(* Logix 5000 AddOnInstructionDefinition export Banner_S15C_MGN_Param_v4; software revision 33.00 *)

TYPE Banner_IOL_Port_v4 :   // UDT that has all of the data items necessary to communicate with a specific Port on a IO-Link Master
STRUCT
   Port_Controlled : INT;   // Each bit represents a port on an IO-Link Master. Set to 1 to tell AOI to control that port.
   Port_Activate : INT;   // Each bit represents a port on an IO-Link Master. When ON that port will process any commands in queue.
   Port_Read : INT;   // Each bit represents a port on an IO-Link Master. Used to determine when device AOI has requested a Read command.
   Port_Write : INT;   // Each bit represents a port on an IO-Link Master. Used to determine when device AOI has requested a Write command.
   Port_RW_Complete : INT;   // Each bit represents a port on an IO-Link Master. Tells device AOI that Read or Write request has been completed.
   Port_Device_Read : INT;
   Data_Transfer : SINT[190];   // Array to transfer data from IO-Master to device AOIs.
END_STRUCT
END_TYPE

TYPE Banner_S15C_MGN_RD_v4 :   // All of the read parameters for a S15C.
STRUCT
   Master_Cycle_Time : INT;
   Min_Cycle_Time : INT;
   M_Sequence_Capability : INT;
   IO_Link_Version_ID : INT;
   Process_Data_Input_Length : INT;
   Process_Data_Output_Length : INT;
   Combined_Vendor_ID : DINT;   // IO-Link Vendor ID
   Vendor_ID1 : INT;
   Vendor_ID2 : INT;
   Combined_Device_ID : DINT;   // IO-Link Device ID
   Device_ID1 : INT;
   Device_ID2 : INT;
   Device_ID3 : INT;
   Serial_Number : STRING;
   Product_Name : STRING;
END_STRUCT
END_TYPE

TYPE Banner_S15C_MGN_v4 :   // All of the parameters for a S15C.
STRUCT
   Initial_Global_Read : BOOL;   // Determines if all of the IO-Link data has been read into the PLC yet
   Command : INT;   // Value placed in here will activate a read or write to a specifc IO-Link Index
   Read : Banner_S15C_MGN_RD_v4;   // Read Only Data
   Write : Banner_S15C_MGN_WD_v4;   // Write Data
   Archive : Banner_S15C_MGN_WD_v4;   // Archive Data
   Reset : BOOL;   // Resets AOI. This will force a complete parameter read of the sensor.
END_STRUCT
END_TYPE

TYPE Banner_S15C_MGN_WD_v4 :   // UDT that stores the Write Data for a S15C.
STRUCT
   System_Command : INT;   // See IODD file for list of commands that can be activated via the System Command interface
   Parameter_Access_Lock : SINT;   // Write access to all parameters is prohibited while value is 1. Only this parameter can be adjusted when value is 1.
   Data_Storage_Lock : SINT;   // Automatic data storage is disabled when this value is equal to 1. Read access is not affected.
   Local_Parameterization_Lock : SINT;   // Parameterization via local control elements on device is disabled.
   Local_User_Interface_Lock : SINT;   // Operation of local user interface is disabled.
   Modbus_Address : DINT;   // 0 to 255
   Modbus_Baud_Rate : DINT;   // 1 to 65535
   Modbus_Parity : DINT;   // 0 to 2
   Modbus_Stop_Bits : DINT;   // 0 to 2
   Modbus_Compliance_Mode : DINT;   // 0 to 4
   RRS : Banner_S15C_RRSS_v4[4];   // Read Register Sets
   WRS : Banner_S15C_WRSS_v4[16];   // Write Registers Set
END_STRUCT
END_TYPE

TYPE Banner_S15C_RRSS_v4 :   // Read Register Set Settings
STRUCT
   MB_Reg : DINT[16];   // Index 1 through 15 are used to store the Modbus Registers
END_STRUCT
END_TYPE

TYPE Banner_S15C_WRSS_v4 :   // Write Register Set Settings
STRUCT
   MB_Reg : DINT;   // Index 1 through 15 are used to store the Modbus registers
   MB_Update_Type : SINT;   // Index 1 through 15 used to store the Modbus registers update type
   MB_Check_Result : SINT;   // Index 1 through 15 used to store the Modbus Check Result
   MB_Write_Cmd_Type : SINT;   // Index 1 through 15 used to store the Write Command type
END_STRUCT
END_TYPE

ADD_ON_INSTRUCTION Banner_S15C_MGN_Param_v4   (* revision 4.0, vendor Banner Engineering *)
// AOI to read and write parameter data to an IO-Link S15C.
VAR_IN_OUT
   S15C : Banner_S15C_MGN_v4; {required}
   Port_Data : Banner_IOL_Port_v4; {required}
END_VAR
VAR_INPUT
   Port : DINT; {required}
END_VAR
VAR
   Local_Control : DINT; {access None}
   Global_Read_Command_Value : INT; {access None}
   Global_Write_Command_Value : INT; {access None}
   Error_Generated : BOOL; {access None}
   Command_Being_Processed : BOOL; {access None}
   Index_Write_Inprocess : INT; {access None}
   Index_Write_Control : INT; {access None}
   Update_Archive : BOOL; {access None}
   Inprocess_Index : DINT; {access None}
   RRS_Index0 : SINT; {access None}
   WRS_Index1 : SINT; {access None}
   WRS_Index0 : SINT; {access None}
   RRS_Index2 : SINT; {access None}
   RRS_Index1 : SINT; {access None}
   RRS_Index3 : SINT; {access None}
   WRS_Index2 : SINT; {access None}
   WRS_Index3 : SINT; {access None}
   WRS_Index4 : SINT; {access None}
   DoNotRun : BOOL; {access None}
   WR_Control : DINT; {access None}
END_VAR

ROUTINE Logic   (* ladder *)
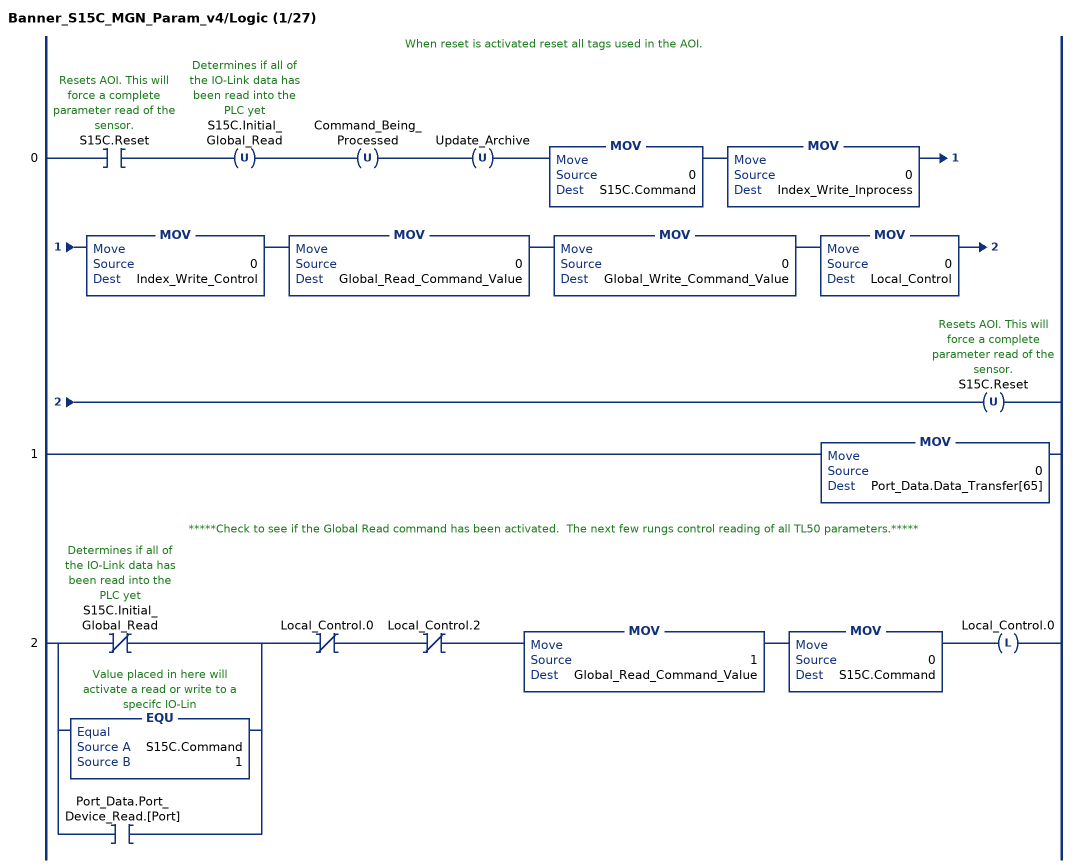
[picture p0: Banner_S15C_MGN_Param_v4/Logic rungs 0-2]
   // When reset is activated reset all tags used in the AOI.
   0: XIC(S15C.Reset)OTU(S15C.Initial_Global_Read)OTU(Command_Being_Processed)OTU(Update_Archive)MOV(0,S15C.Command)MOV(0,Index_Write_Inprocess)MOV(0,Index_Write_Control)MOV(0,Global_Read_Command_Value)MOV(0,Global_Write_Command_Value)MOV(0,Local_Control)OTU(S15C.Reset);
   1: MOV(0,Port_Data.Data_Transfer[65]);
   // *****Check to see if the Global Read command has been activated.  The next few rungs control reading of all TL50 parameters.*****
   2: [XIO(S15C.Initial_Global_Read) ,EQU(S15C.Command,1) ,XIC(Port_Data.Port_Device_Read.[Port]) ]XIO(Local_Control.0)XIO(Local_Control.2)MOV(1,Global_Read_Command_Value)MOV(0,S15C.Command)OTL(Local_Control.0);
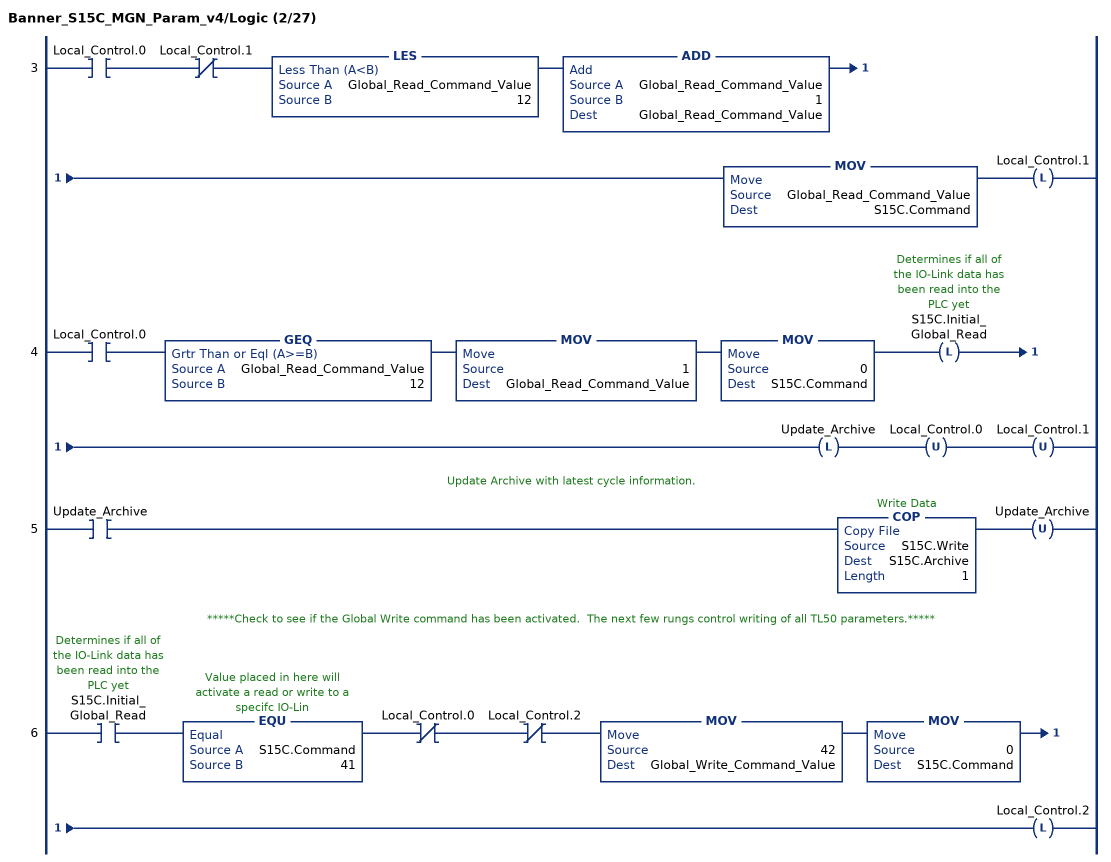
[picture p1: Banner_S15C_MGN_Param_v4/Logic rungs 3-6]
   3: XIC(Local_Control.0)XIO(Local_Control.1)LES(Global_Read_Command_Value,12)ADD(Global_Read_Command_Value,1,Global_Read_Command_Value)MOV(Global_Read_Command_Value,S15C.Command)OTL(Local_Control.1);
   4: XIC(Local_Control.0)GEQ(Global_Read_Command_Value,12)MOV(1,Global_Read_Command_Value)MOV(0,S15C.Command)OTL(S15C.Initial_Global_Read)OTL(Update_Archive)OTU(Local_Control.0)OTU(Local_Control.1);
   // Update Archive with latest cycle information.
   5: XIC(Update_Archive)COP(S15C.Write,S15C.Archive,1)OTU(Update_Archive);
   // *****Check to see if the Global Write command has been activated.  The next few rungs control writing of all TL50 parameters.*****
   6: XIC(S15C.Initial_Global_Read)EQU(S15C.Command,41)XIO(Local_Control.0)XIO(Local_Control.2)MOV(42,Global_Write_Command_Value)MOV(0,S15C.Command)OTL(Local_Control.2);
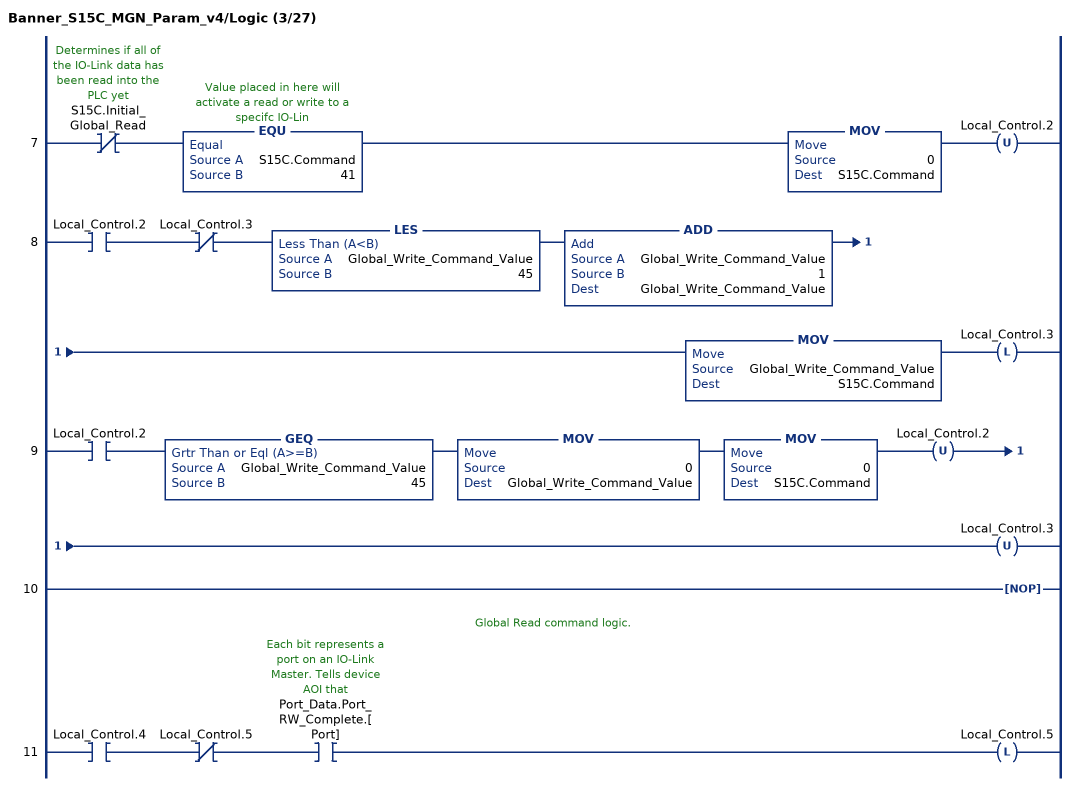
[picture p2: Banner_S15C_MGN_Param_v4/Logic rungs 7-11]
   7: XIO(S15C.Initial_Global_Read)EQU(S15C.Command,41)MOV(0,S15C.Command)OTU(Local_Control.2);
   8: XIC(Local_Control.2)XIO(Local_Control.3)LES(Global_Write_Command_Value,45)ADD(Global_Write_Command_Value,1,Global_Write_Command_Value)MOV(Global_Write_Command_Value,S15C.Command)OTL(Local_Control.3);
   9: XIC(Local_Control.2)GEQ(Global_Write_Command_Value,45)MOV(0,Global_Write_Command_Value)MOV(0,S15C.Command)OTU(Local_Control.2)OTU(Local_Control.3);
   10: NOP();
   // Global Read command logic.
   11: XIC(Local_Control.4)XIO(Local_Control.5)XIC(Port_Data.Port_RW_Complete.[Port])OTL(Local_Control.5);
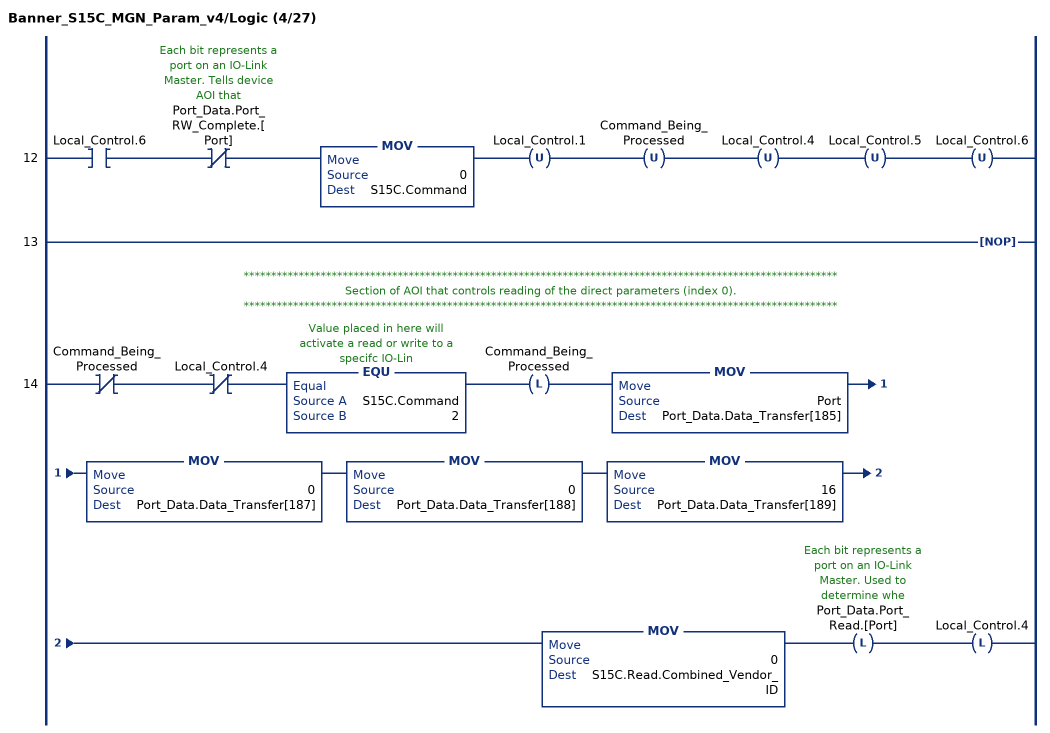
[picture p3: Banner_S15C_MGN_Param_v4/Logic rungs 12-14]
   12: XIC(Local_Control.6)XIO(Port_Data.Port_RW_Complete.[Port])MOV(0,S15C.Command)OTU(Local_Control.1)OTU(Command_Being_Processed)OTU(Local_Control.4)OTU(Local_Control.5)OTU(Local_Control.6);
   13: NOP();
   // ************************************************************************************************************
   // Section of AOI that controls reading of the direct parameters (index 0).
   // ************************************************************************************************************
   14: XIO(Command_Being_Processed)XIO(Local_Control.4)EQU(S15C.Command,2)OTL(Command_Being_Processed)MOV(Port,Port_Data.Data_Transfer[185])MOV(0,Port_Data.Data_Transfer[187])MOV(0,Port_Data.Data_Transfer[188])MOV(16,Port_Data.Data_Transfer[189])MOV(0,S15C.Read.Combined_Vendor_ID)OTL(Port_Data.Port_Read.[Port])OTL(Local_Control.4);
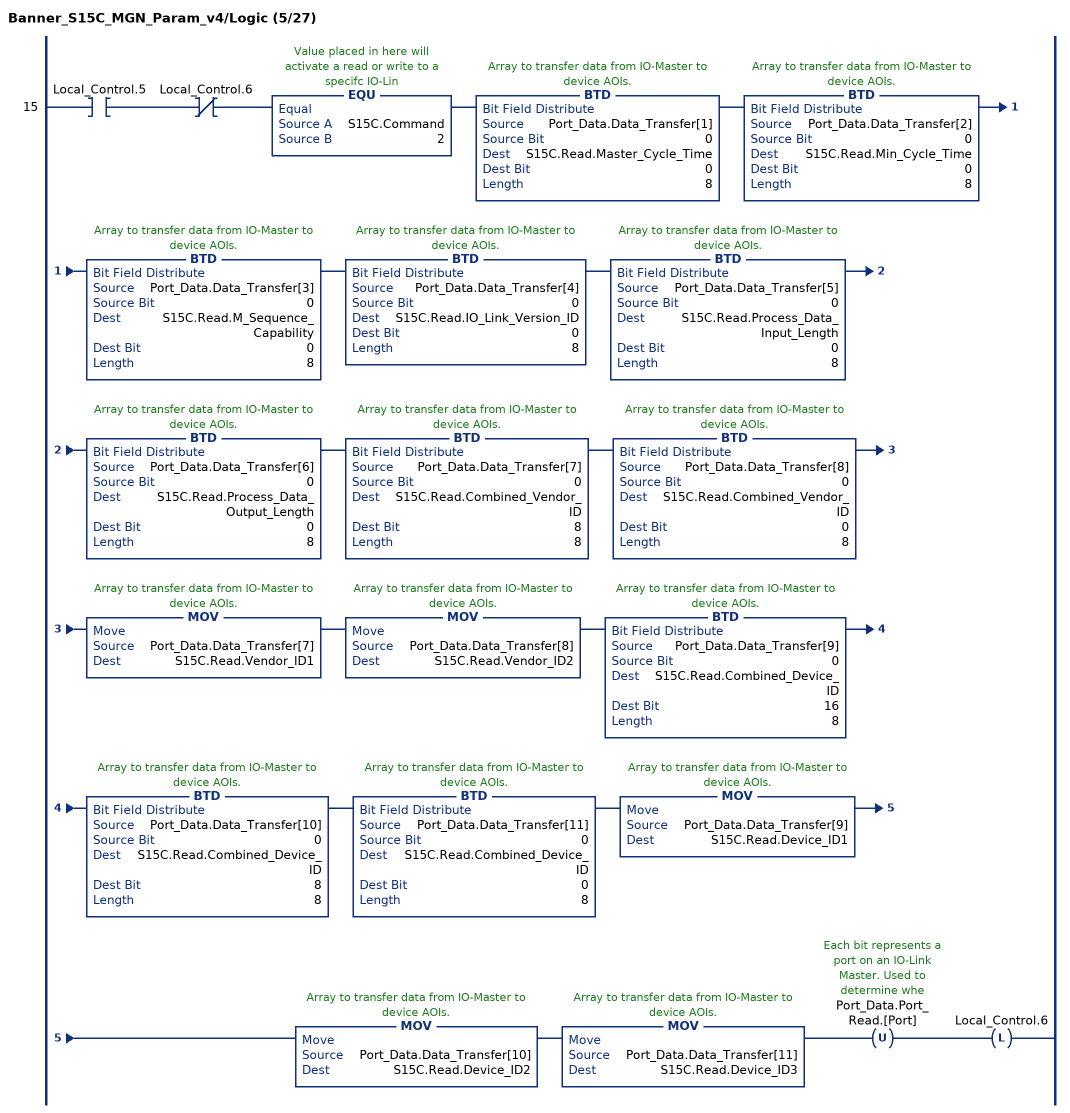
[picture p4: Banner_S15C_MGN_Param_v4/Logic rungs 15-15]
   15: XIC(Local_Control.5)XIO(Local_Control.6)EQU(S15C.Command,2)BTD(Port_Data.Data_Transfer[1],0,S15C.Read.Master_Cycle_Time,0,8)BTD(Port_Data.Data_Transfer[2],0,S15C.Read.Min_Cycle_Time,0,8)BTD(Port_Data.Data_Transfer[3],0,S15C.Read.M_Sequence_Capability,0,8)BTD(Port_Data.Data_Transfer[4],0,S15C.Read.IO_Link_Version_ID,0,8)BTD(Port_Data.Data_Transfer[5],0,S15C.Read.Process_Data_Input_Length,0,8)BTD(Port_Data.Data_Transfer[6],0,S15C.Read.Process_Data_Output_Length,0,8)BTD(Port_Data.Data_Transfer[7],0,S15C.Read.Combined_Vendor_ID,8,8)BTD(Port_Data.Data_Transfer[8],0,S15C.Read.Combined_Vendor_ID,0,8)MOV(Port_Data.Data_Transfer[7],S15C.Read.Vendor_ID1)MOV(Port_Data.Data_Transfer[8],S15C.Read.Vendor_ID2)BTD(Port_Data.Data_Transfer[9],0,S15C.Read.Combined_Device_ID,16,8)BTD(Port_Data.Data_Transfer[10],0,S15C.Read.Combined_Device_ID,8,8)BTD(Port_Data.Data_Transfer[11],0,S15C.Read.Combined_Device_ID,0,8)MOV(Port_Data.Data_Transfer[9],S15C.Read.Device_ID1)MOV(Port_Data.Data_Transfer[10],S15C.Read.Device_ID2)MOV(Port_Data.Data_Transfer[11],S15C.Read.Device_ID3)OTU(Port_Data.Port_Read.[Port])OTL(Local_Control.6);
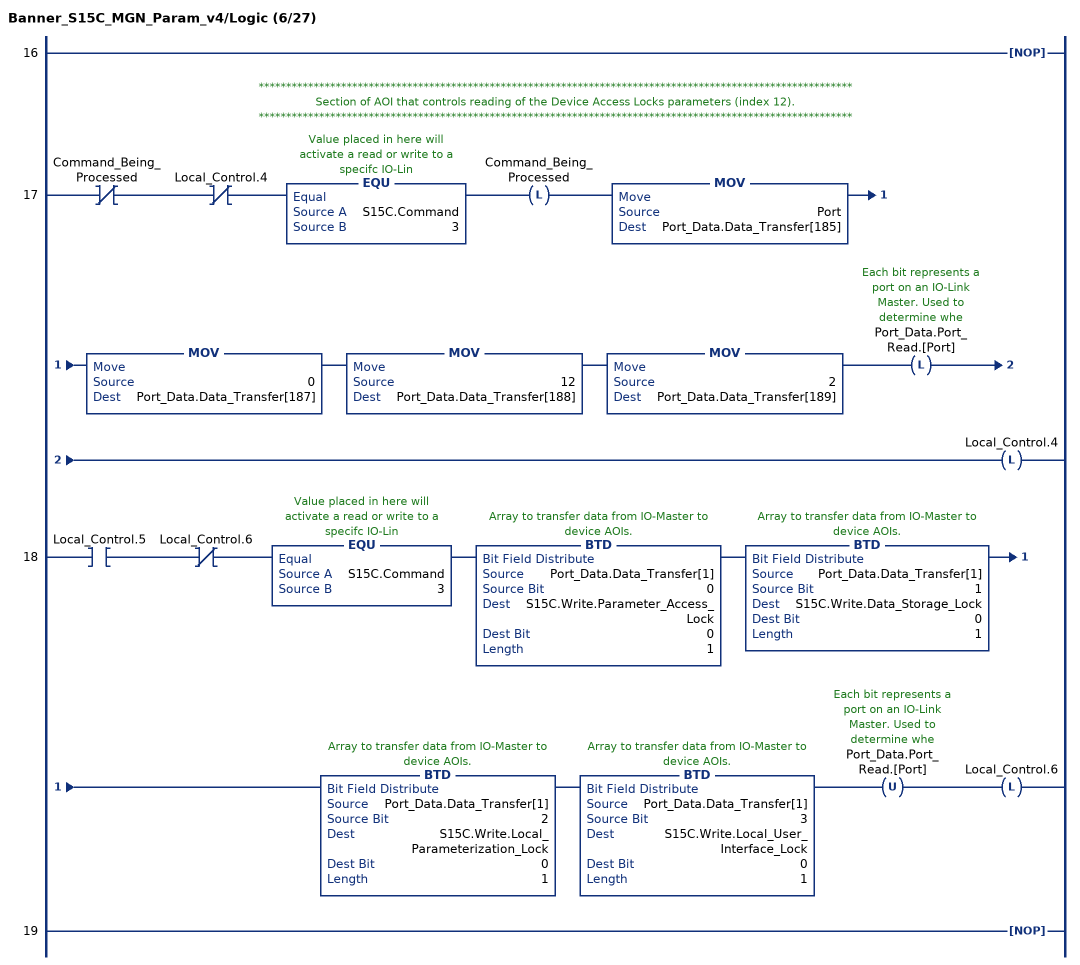
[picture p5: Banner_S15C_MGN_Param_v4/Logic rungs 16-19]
   16: NOP();
   // ************************************************************************************************************
   // Section of AOI that controls reading of the Device Access Locks parameters (index 12).
   // ************************************************************************************************************
   17: XIO(Command_Being_Processed)XIO(Local_Control.4)EQU(S15C.Command,3)OTL(Command_Being_Processed)MOV(Port,Port_Data.Data_Transfer[185])MOV(0,Port_Data.Data_Transfer[187])MOV(12,Port_Data.Data_Transfer[188])MOV(2,Port_Data.Data_Transfer[189])OTL(Port_Data.Port_Read.[Port])OTL(Local_Control.4);
   18: XIC(Local_Control.5)XIO(Local_Control.6)EQU(S15C.Command,3)BTD(Port_Data.Data_Transfer[1],0,S15C.Write.Parameter_Access_Lock,0,1)BTD(Port_Data.Data_Transfer[1],1,S15C.Write.Data_Storage_Lock,0,1)BTD(Port_Data.Data_Transfer[1],2,S15C.Write.Local_Parameterization_Lock,0,1)BTD(Port_Data.Data_Transfer[1],3,S15C.Write.Local_User_Interface_Lock,0,1)OTU(Port_Data.Port_Read.[Port])OTL(Local_Control.6);
   19: NOP();
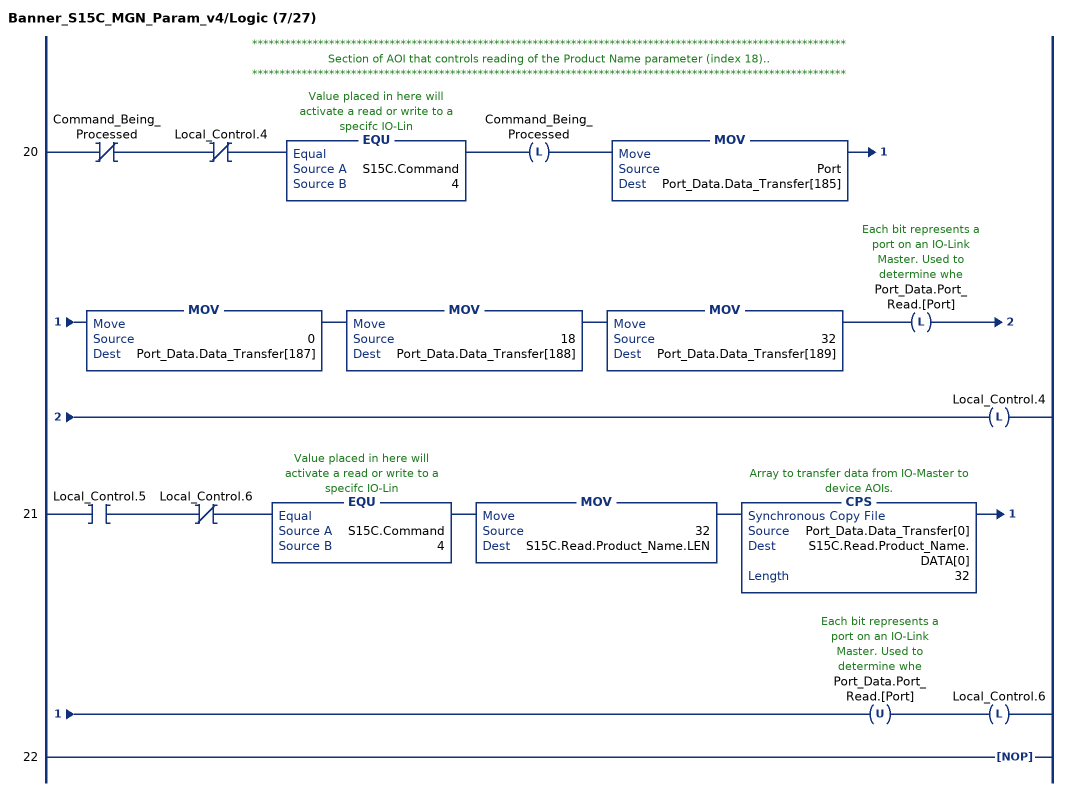
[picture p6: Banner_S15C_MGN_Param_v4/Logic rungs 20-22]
   // ************************************************************************************************************
   // Section of AOI that controls reading of the Product Name parameter (index 18)..
   // ************************************************************************************************************
   20: XIO(Command_Being_Processed)XIO(Local_Control.4)EQU(S15C.Command,4)OTL(Command_Being_Processed)MOV(Port,Port_Data.Data_Transfer[185])MOV(0,Port_Data.Data_Transfer[187])MOV(18,Port_Data.Data_Transfer[188])MOV(32,Port_Data.Data_Transfer[189])OTL(Port_Data.Port_Read.[Port])OTL(Local_Control.4);
   21: XIC(Local_Control.5)XIO(Local_Control.6)EQU(S15C.Command,4)MOV(32,S15C.Read.Product_Name.LEN)CPS(Port_Data.Data_Transfer[0],S15C.Read.Product_Name.DATA[0],32)OTU(Port_Data.Port_Read.[Port])OTL(Local_Control.6);
   22: NOP();
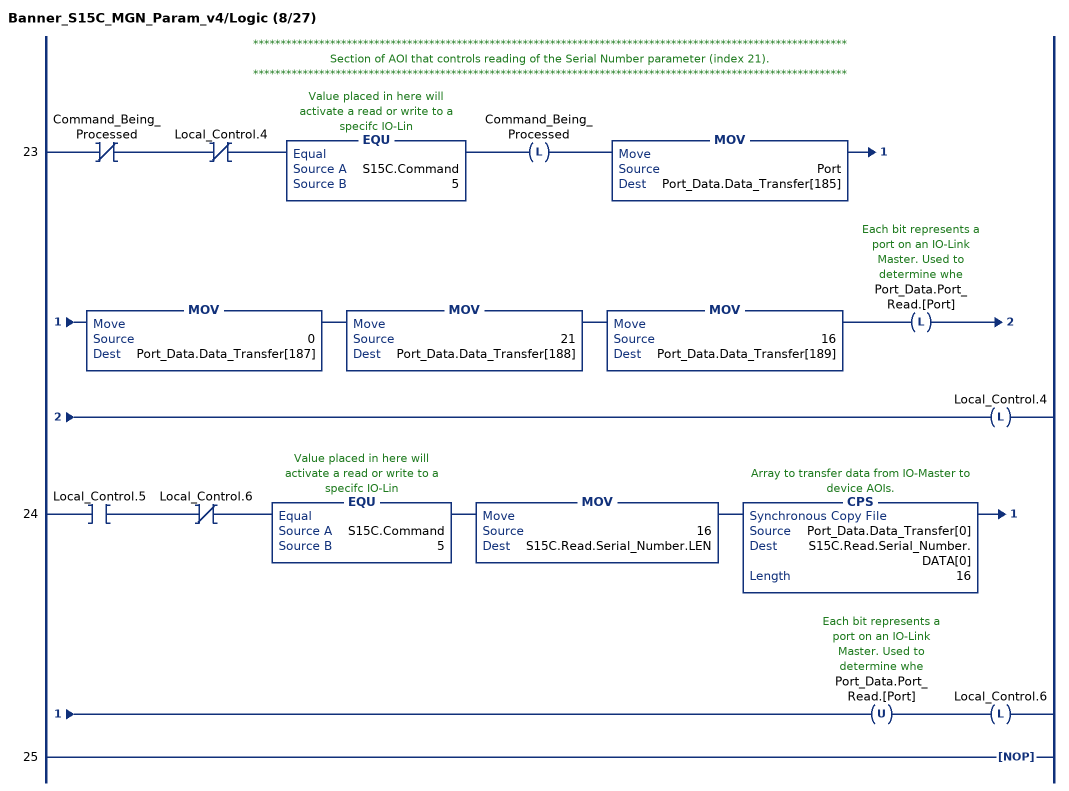
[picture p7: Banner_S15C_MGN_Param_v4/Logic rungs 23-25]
   // ************************************************************************************************************
   // Section of AOI that controls reading of the Serial Number parameter (index 21).
   // ************************************************************************************************************
   23: XIO(Command_Being_Processed)XIO(Local_Control.4)EQU(S15C.Command,5)OTL(Command_Being_Processed)MOV(Port,Port_Data.Data_Transfer[185])MOV(0,Port_Data.Data_Transfer[187])MOV(21,Port_Data.Data_Transfer[188])MOV(16,Port_Data.Data_Transfer[189])OTL(Port_Data.Port_Read.[Port])OTL(Local_Control.4);
   24: XIC(Local_Control.5)XIO(Local_Control.6)EQU(S15C.Command,5)MOV(16,S15C.Read.Serial_Number.LEN)CPS(Port_Data.Data_Transfer[0],S15C.Read.Serial_Number.DATA[0],16)OTU(Port_Data.Port_Read.[Port])OTL(Local_Control.6);
   25: NOP();
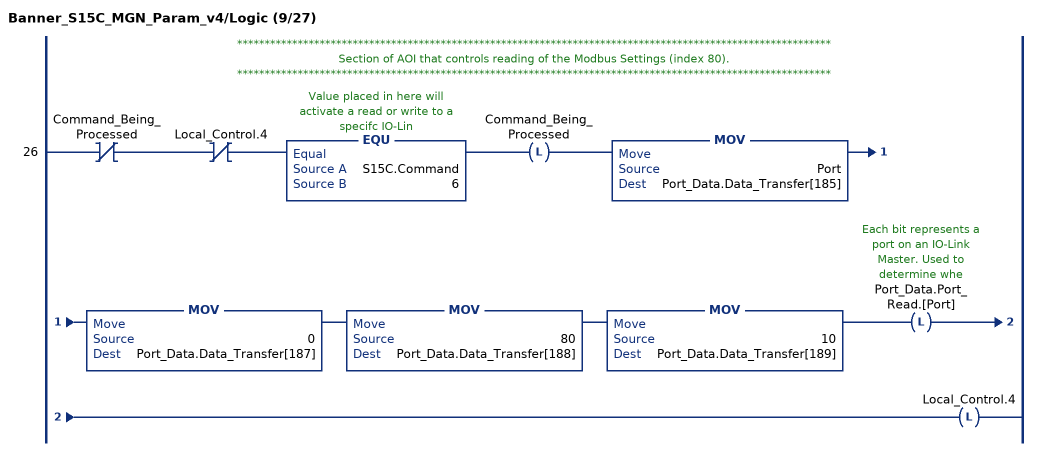
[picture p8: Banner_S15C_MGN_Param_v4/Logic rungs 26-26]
   // ************************************************************************************************************
   // Section of AOI that controls reading of the Modbus Settings (index 80).
   // ************************************************************************************************************
   26: XIO(Command_Being_Processed)XIO(Local_Control.4)EQU(S15C.Command,6)OTL(Command_Being_Processed)MOV(Port,Port_Data.Data_Transfer[185])MOV(0,Port_Data.Data_Transfer[187])MOV(80,Port_Data.Data_Transfer[188])MOV(10,Port_Data.Data_Transfer[189])OTL(Port_Data.Port_Read.[Port])OTL(Local_Control.4);
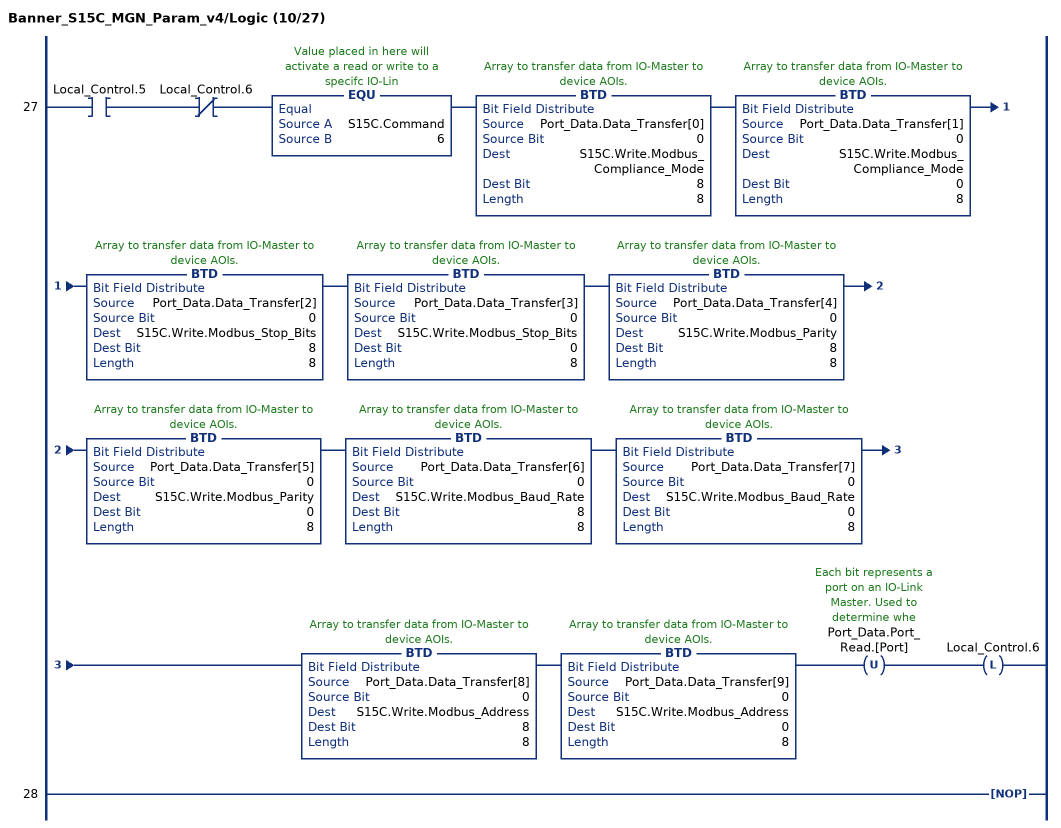
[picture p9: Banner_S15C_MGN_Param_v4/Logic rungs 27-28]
   27: XIC(Local_Control.5)XIO(Local_Control.6)EQU(S15C.Command,6)BTD(Port_Data.Data_Transfer[0],0,S15C.Write.Modbus_Compliance_Mode,8,8)BTD(Port_Data.Data_Transfer[1],0,S15C.Write.Modbus_Compliance_Mode,0,8)BTD(Port_Data.Data_Transfer[2],0,S15C.Write.Modbus_Stop_Bits,8,8)BTD(Port_Data.Data_Transfer[3],0,S15C.Write.Modbus_Stop_Bits,0,8)BTD(Port_Data.Data_Transfer[4],0,S15C.Write.Modbus_Parity,8,8)BTD(Port_Data.Data_Transfer[5],0,S15C.Write.Modbus_Parity,0,8)BTD(Port_Data.Data_Transfer[6],0,S15C.Write.Modbus_Baud_Rate,8,8)BTD(Port_Data.Data_Transfer[7],0,S15C.Write.Modbus_Baud_Rate,0,8)BTD(Port_Data.Data_Transfer[8],0,S15C.Write.Modbus_Address,8,8)BTD(Port_Data.Data_Transfer[9],0,S15C.Write.Modbus_Address,0,8)OTU(Port_Data.Port_Read.[Port])OTL(Local_Control.6);
   28: NOP();
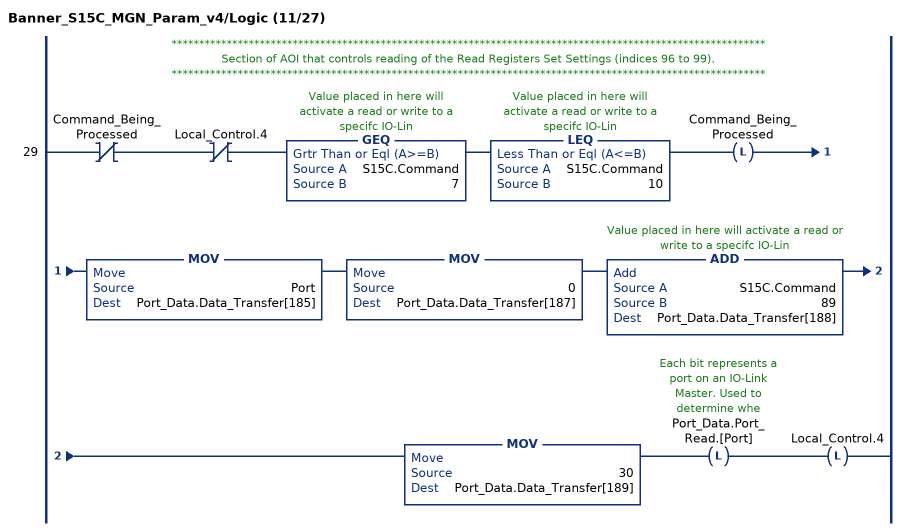
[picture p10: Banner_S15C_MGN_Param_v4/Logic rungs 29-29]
   // ************************************************************************************************************
   // Section of AOI that controls reading of the Read Registers Set Settings (indices 96 to 99).
   // ************************************************************************************************************
   29: XIO(Command_Being_Processed)XIO(Local_Control.4)GEQ(S15C.Command,7)LEQ(S15C.Command,10)OTL(Command_Being_Processed)MOV(Port,Port_Data.Data_Transfer[185])MOV(0,Port_Data.Data_Transfer[187])ADD(S15C.Command,89,Port_Data.Data_Transfer[188])MOV(30,Port_Data.Data_Transfer[189])OTL(Port_Data.Port_Read.[Port])OTL(Local_Control.4);
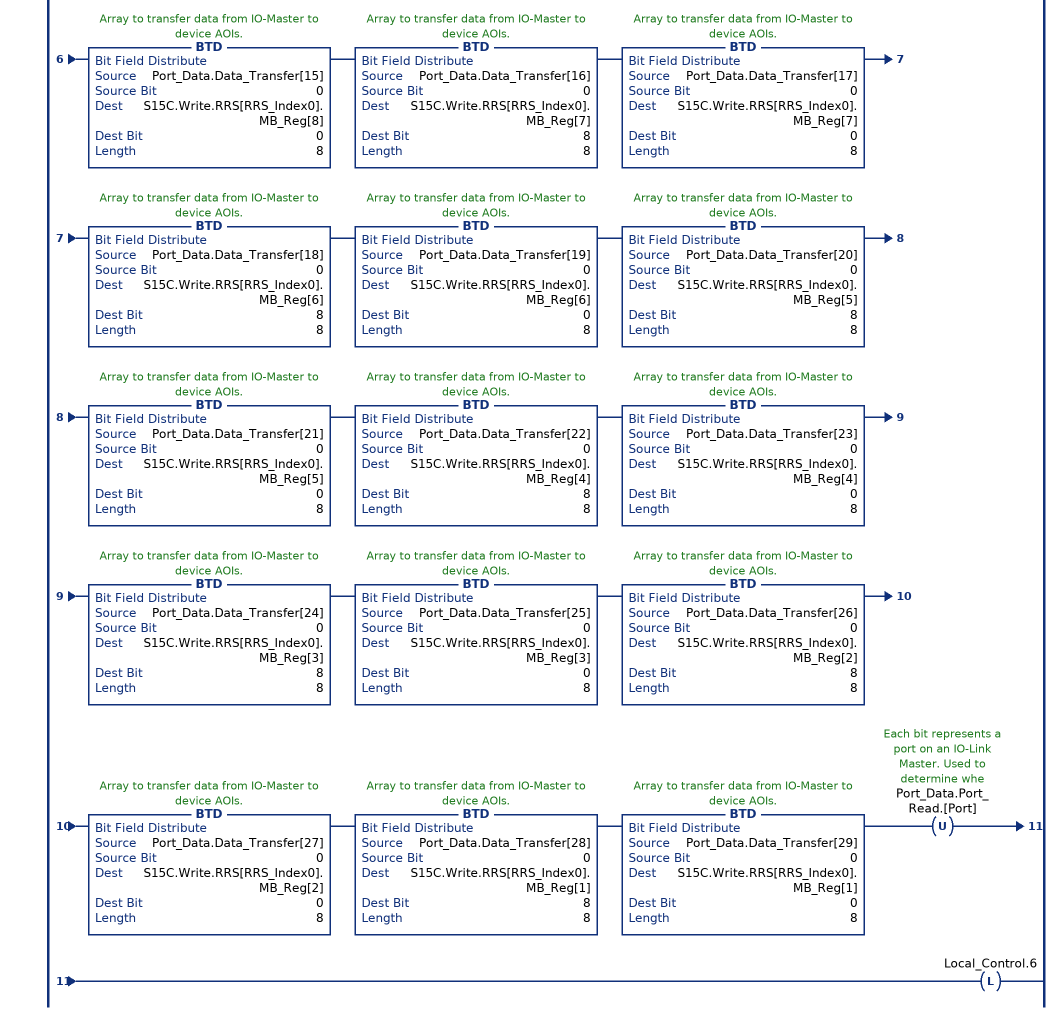
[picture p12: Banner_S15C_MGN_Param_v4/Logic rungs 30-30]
   30: XIC(Local_Control.5)XIO(Local_Control.6)GEQ(S15C.Command,7)LEQ(S15C.Command,10)SUB(S15C.Command,7,RRS_Index0)BTD(Port_Data.Data_Transfer[0],0,S15C.Write.RRS[RRS_Index0].MB_Reg[15],8,8)BTD(Port_Data.Data_Transfer[1],0,S15C.Write.RRS[RRS_Index0].MB_Reg[15],0,8)BTD(Port_Data.Data_Transfer[2],0,S15C.Write.RRS[RRS_Index0].MB_Reg[14],8,8)BTD(Port_Data.Data_Transfer[3],0,S15C.Write.RRS[RRS_Index0].MB_Reg[14],0,8)BTD(Port_Data.Data_Transfer[4],0,S15C.Write.RRS[RRS_Index0].MB_Reg[13],8,8)BTD(Port_Data.Data_Transfer[5],0,S15C.Write.RRS[RRS_Index0].MB_Reg[13],0,8)BTD(Port_Data.Data_Transfer[6],0,S15C.Write.RRS[RRS_Index0].MB_Reg[12],8,8)BTD(Port_Data.Data_Transfer[7],0,S15C.Write.RRS[RRS_Index0].MB_Reg[12],0,8)BTD(Port_Data.Data_Transfer[8],0,S15C.Write.RRS[RRS_Index0].MB_Reg[11],8,8)BTD(Port_Data.Data_Transfer[9],0,S15C.Write.RRS[RRS_Index0].MB_Reg[11],0,8)BTD(Port_Data.Data_Transfer[10],0,S15C.Write.RRS[RRS_Index0].MB_Reg[10],8,8)BTD(Port_Data.Data_Transfer[11],0,S15C.Write.RRS[RRS_Index0].MB_Reg[10],0,8)BTD(Port_Data.Data_Transfer[12],0,S15C.Write.RRS[RRS_Index0].MB_Reg[9],8,8)BTD(Port_Data.Data_Transfer[13],0,S15C.Write.RRS[RRS_Index0].MB_Reg[9],0,8)BTD(Port_Data.Data_Transfer[14],0,S15C.Write.RRS[RRS_Index0].MB_Reg[8],8,8)BTD(Port_Data.Data_Transfer[15],0,S15C.Write.RRS[RRS_Index0].MB_Reg[8],0,8)BTD(Port_Data.Data_Transfer[16],0,S15C.Write.RRS[RRS_Index0].MB_Reg[7],8,8)BTD(Port_Data.Data_Transfer[17],0,S15C.Write.RRS[RRS_Index0].MB_Reg[7],0,8)BTD(Port_Data.Data_Transfer[18],0,S15C.Write.RRS[RRS_Index0].MB_Reg[6],8,8)BTD(Port_Data.Data_Transfer[19],0,S15C.Write.RRS[RRS_Index0].MB_Reg[6],0,8)BTD(Port_Data.Data_Transfer[20],0,S15C.Write.RRS[RRS_Index0].MB_Reg[5],8,8)BTD(Port_Data.Data_Transfer[21],0,S15C.Write.RRS[RRS_Index0].MB_Reg[5],0,8)BTD(Port_Data.Data_Transfer[22],0,S15C.Write.RRS[RRS_Index0].MB_Reg[4],8,8)BTD(Port_Data.Data_Transfer[23],0,S15C.Write.RRS[RRS_Index0].MB_Reg[4],0,8)BTD(Port_Data.Data_Transfer[24],0,S15C.Write.RRS[RRS_Index0].MB_Reg[3],8,8)BTD(Port_Data.Data_Transfer[25],0,S15C.Write.RRS[RRS_Index0].MB_Reg[3],0,8)BTD(Port_Data.Data_Transfer[26],0,S15C.Write.RRS[RRS_Index0].MB_Reg[2],8,8)BTD(Port_Data.Data_Transfer[27],0,S15C.Write.RRS[RRS_Index0].MB_Reg[2],0,8)BTD(Port_Data.Data_Transfer[28],0,S15C.Write.RRS[RRS_Index0].MB_Reg[1],8,8)BTD(Port_Data.Data_Transfer[29],0,S15C.Write.RRS[RRS_Index0].MB_Reg[1],0,8)OTU(Port_Data.Port_Read.[Port])OTL(Local_Control.6);
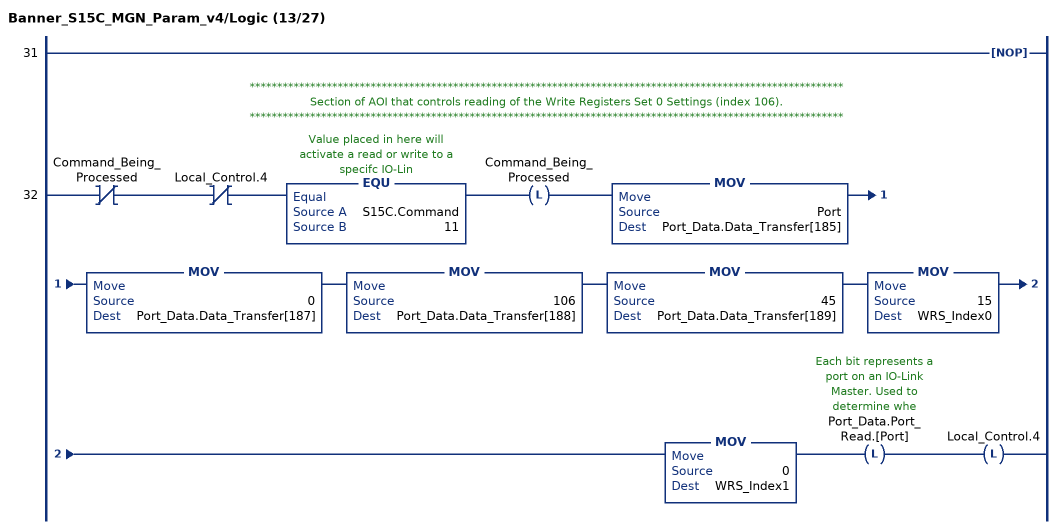
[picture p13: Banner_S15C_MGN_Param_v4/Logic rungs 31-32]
   31: NOP();
   // ************************************************************************************************************
   // Section of AOI that controls reading of the Write Registers Set 0 Settings (index 106).
   // ************************************************************************************************************
   32: XIO(Command_Being_Processed)XIO(Local_Control.4)EQU(S15C.Command,11)OTL(Command_Being_Processed)MOV(Port,Port_Data.Data_Transfer[185])MOV(0,Port_Data.Data_Transfer[187])MOV(106,Port_Data.Data_Transfer[188])MOV(45,Port_Data.Data_Transfer[189])MOV(15,WRS_Index0)MOV(0,WRS_Index1)OTL(Port_Data.Port_Read.[Port])OTL(Local_Control.4);
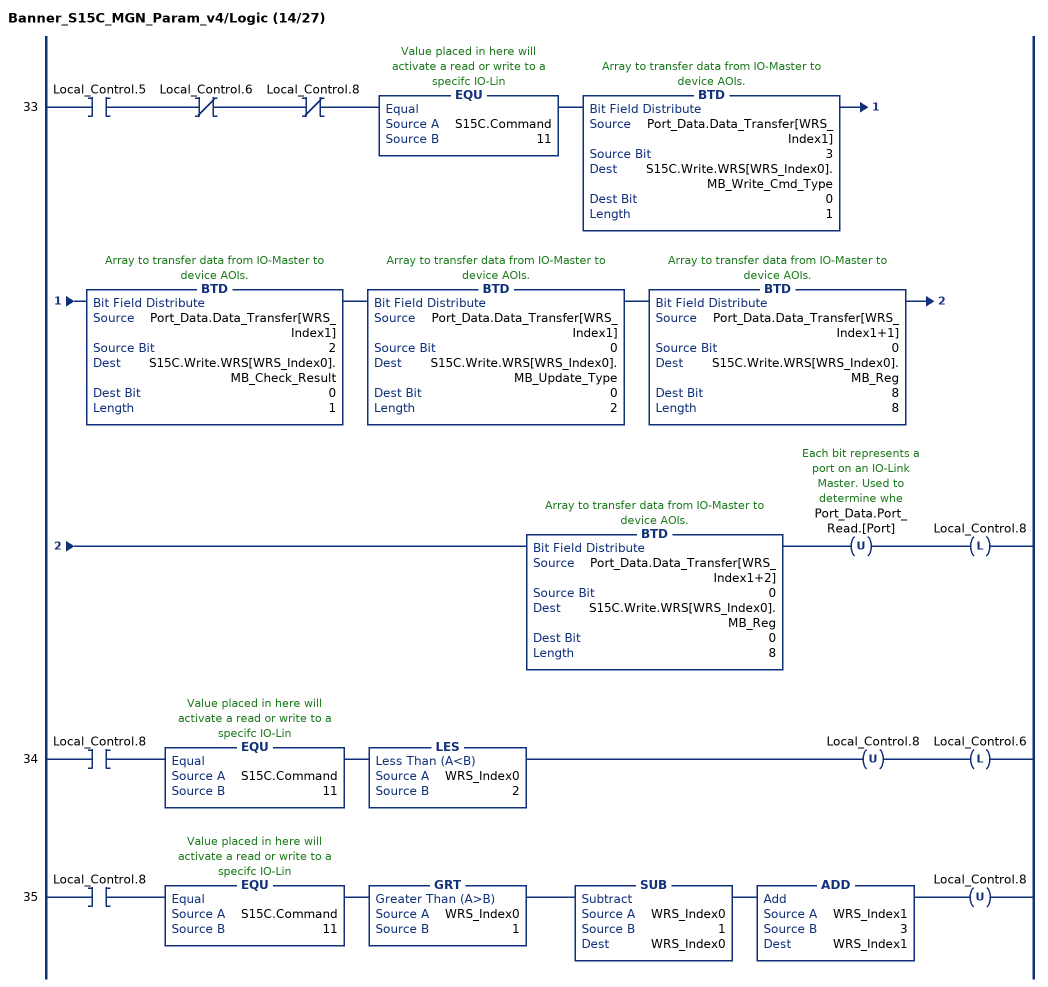
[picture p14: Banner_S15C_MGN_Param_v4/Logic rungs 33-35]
   33: XIC(Local_Control.5)XIO(Local_Control.6)XIO(Local_Control.8)EQU(S15C.Command,11)BTD(Port_Data.Data_Transfer[WRS_Index1],3,S15C.Write.WRS[WRS_Index0].MB_Write_Cmd_Type,0,1)BTD(Port_Data.Data_Transfer[WRS_Index1],2,S15C.Write.WRS[WRS_Index0].MB_Check_Result,0,1)BTD(Port_Data.Data_Transfer[WRS_Index1],0,S15C.Write.WRS[WRS_Index0].MB_Update_Type,0,2)BTD(Port_Data.Data_Transfer[WRS_Index1+1],0,S15C.Write.WRS[WRS_Index0].MB_Reg,8,8)BTD(Port_Data.Data_Transfer[WRS_Index1+2],0,S15C.Write.WRS[WRS_Index0].MB_Reg,0,8)OTU(Port_Data.Port_Read.[Port])OTL(Local_Control.8);
   34: XIC(Local_Control.8)EQU(S15C.Command,11)LES(WRS_Index0,2)OTU(Local_Control.8)OTL(Local_Control.6);
   35: XIC(Local_Control.8)EQU(S15C.Command,11)GRT(WRS_Index0,1)SUB(WRS_Index0,1,WRS_Index0)ADD(WRS_Index1,3,WRS_Index1)OTU(Local_Control.8);
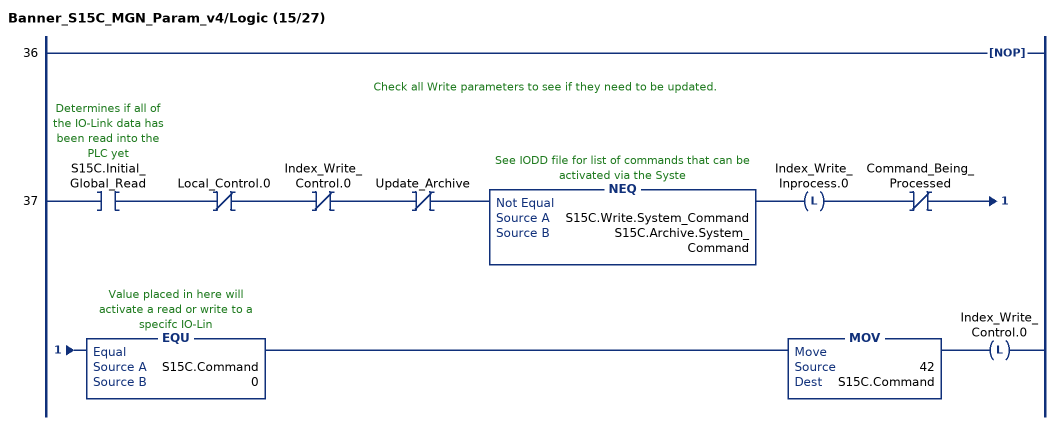
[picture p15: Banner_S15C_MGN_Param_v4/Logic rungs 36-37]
   36: NOP();
   // Check all Write parameters to see if they need to be updated.
   37: XIC(S15C.Initial_Global_Read)XIO(Local_Control.0)XIO(Index_Write_Control.0)XIO(Update_Archive)NEQ(S15C.Write.System_Command,S15C.Archive.System_Command)OTL(Index_Write_Inprocess.0)XIO(Command_Being_Processed)EQU(S15C.Command,0)MOV(42,S15C.Command)OTL(Index_Write_Control.0);
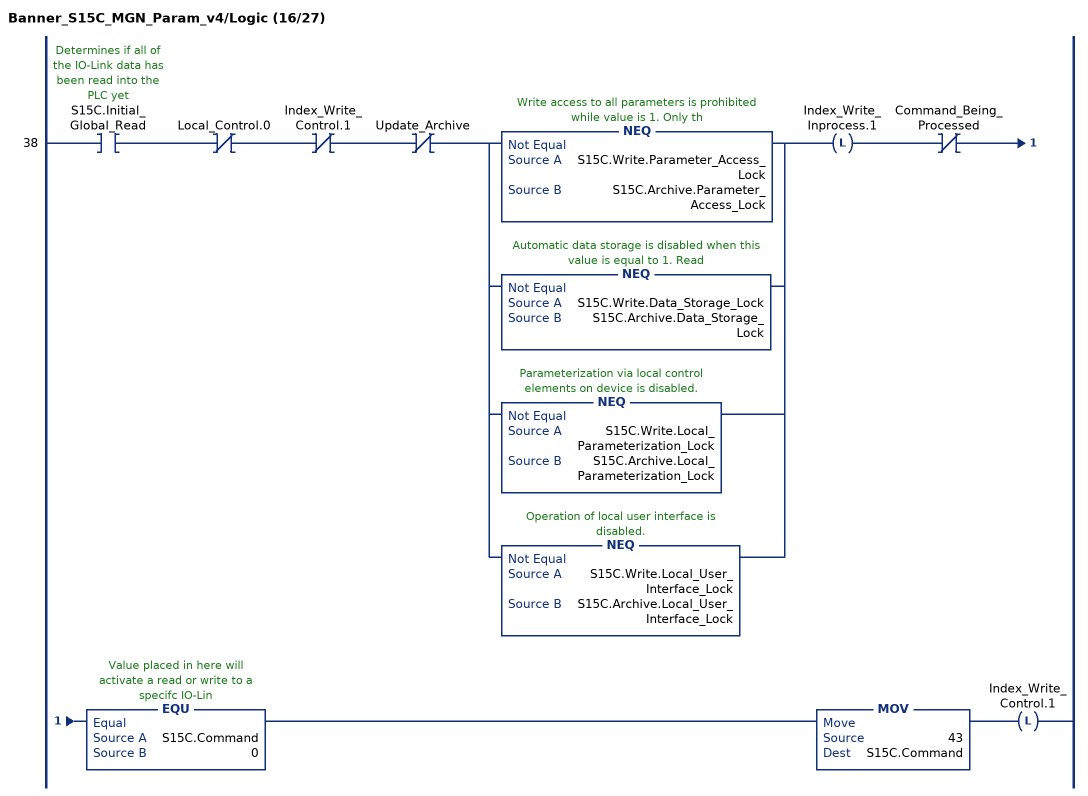
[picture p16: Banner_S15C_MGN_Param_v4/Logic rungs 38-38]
   38: XIC(S15C.Initial_Global_Read)XIO(Local_Control.0)XIO(Index_Write_Control.1)XIO(Update_Archive)[NEQ(S15C.Write.Parameter_Access_Lock,S15C.Archive.Parameter_Access_Lock) ,NEQ(S15C.Write.Data_Storage_Lock,S15C.Archive.Data_Storage_Lock) ,NEQ(S15C.Write.Local_Parameterization_Lock,S15C.Archive.Local_Parameterization_Lock) ,NEQ(S15C.Write.Local_User_Interface_Lock,S15C.Archive.Local_User_Interface_Lock) ]OTL(Index_Write_Inprocess.1)XIO(Command_Being_Processed)EQU(S15C.Command,0)MOV(43,S15C.Command)OTL(Index_Write_Control.1);
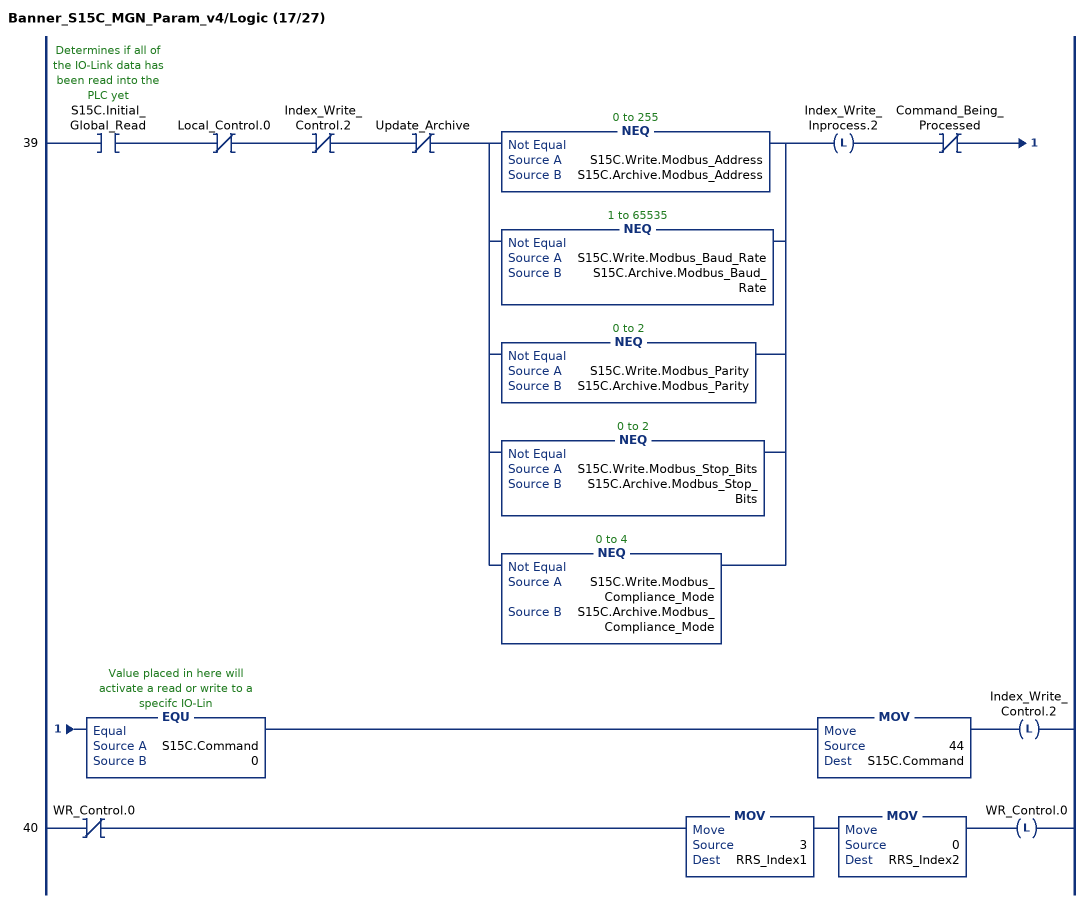
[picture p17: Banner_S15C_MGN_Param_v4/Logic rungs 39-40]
   39: XIC(S15C.Initial_Global_Read)XIO(Local_Control.0)XIO(Index_Write_Control.2)XIO(Update_Archive)[NEQ(S15C.Write.Modbus_Address,S15C.Archive.Modbus_Address) ,NEQ(S15C.Write.Modbus_Baud_Rate,S15C.Archive.Modbus_Baud_Rate) ,NEQ(S15C.Write.Modbus_Parity,S15C.Archive.Modbus_Parity) ,NEQ(S15C.Write.Modbus_Stop_Bits,S15C.Archive.Modbus_Stop_Bits) ,NEQ(S15C.Write.Modbus_Compliance_Mode,S15C.Archive.Modbus_Compliance_Mode) ]OTL(Index_Write_Inprocess.2)XIO(Command_Being_Processed)EQU(S15C.Command,0)MOV(44,S15C.Command)OTL(Index_Write_Control.2);
   40: XIO(WR_Control.0)MOV(3,RRS_Index1)MOV(0,RRS_Index2)OTL(WR_Control.0);
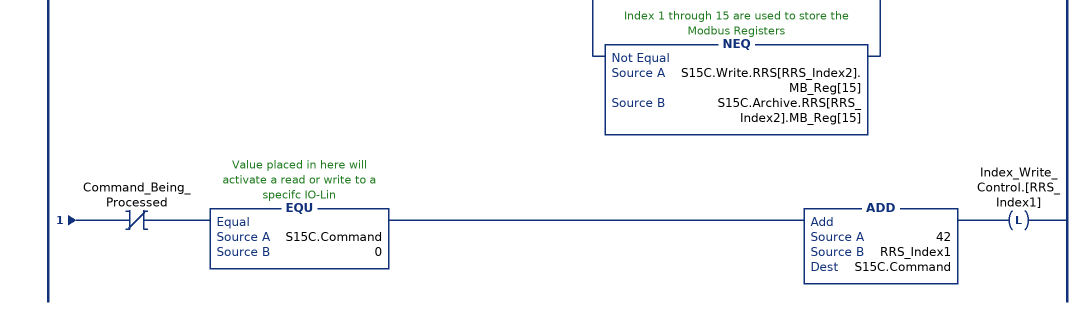
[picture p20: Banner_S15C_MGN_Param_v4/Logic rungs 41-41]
   41: XIC(S15C.Initial_Global_Read)XIC(WR_Control.0)XIO(Local_Control.0)XIO(Index_Write_Control.[RRS_Index1])XIO(Update_Archive)[NEQ(S15C.Write.RRS[RRS_Index2].MB_Reg[1],S15C.Archive.RRS[RRS_Index2].MB_Reg[1]) ,NEQ(S15C.Write.RRS[RRS_Index2].MB_Reg[2],S15C.Archive.RRS[RRS_Index2].MB_Reg[2]) ,NEQ(S15C.Write.RRS[RRS_Index2].MB_Reg[3],S15C.Archive.RRS[RRS_Index2].MB_Reg[3]) ,NEQ(S15C.Write.RRS[RRS_Index2].MB_Reg[4],S15C.Archive.RRS[RRS_Index2].MB_Reg[4]) ,NEQ(S15C.Write.RRS[RRS_Index2].MB_Reg[5],S15C.Archive.RRS[RRS_Index2].MB_Reg[5]) ,NEQ(S15C.Write.RRS[RRS_Index2].MB_Reg[6],S15C.Archive.RRS[RRS_Index2].MB_Reg[6]) ,NEQ(S15C.Write.RRS[RRS_Index2].MB_Reg[7],S15C.Archive.RRS[RRS_Index2].MB_Reg[7]) ,NEQ(S15C.Write.RRS[RRS_Index2].MB_Reg[8],S15C.Archive.RRS[RRS_Index2].MB_Reg[8]) ,NEQ(S15C.Write.RRS[RRS_Index2].MB_Reg[9],S15C.Archive.RRS[RRS_Index2].MB_Reg[9]) ,NEQ(S15C.Write.RRS[RRS_Index2].MB_Reg[10],S15C.Archive.RRS[RRS_Index2].MB_Reg[10]) ,NEQ(S15C.Write.RRS[RRS_Index2].MB_Reg[11],S15C.Archive.RRS[RRS_Index2].MB_Reg[11]) ,NEQ(S15C.Write.RRS[RRS_Index2].MB_Reg[12],S15C.Archive.RRS[RRS_Index2].MB_Reg[12]) ,NEQ(S15C.Write.RRS[RRS_Index2].MB_Reg[13],S15C.Archive.RRS[RRS_Index2].MB_Reg[13]) ,NEQ(S15C.Write.RRS[RRS_Index2].MB_Reg[14],S15C.Archive.RRS[RRS_Index2].MB_Reg[14]) ,NEQ(S15C.Write.RRS[RRS_Index2].MB_Reg[15],S15C.Archive.RRS[RRS_Index2].MB_Reg[15]) ]OTL(Index_Write_Inprocess.[RRS_Index1])XIO(Command_Being_Processed)EQU(S15C.Command,0)ADD(42,RRS_Index1,S15C.Command)OTL(Index_Write_Control.[RRS_Index1]);
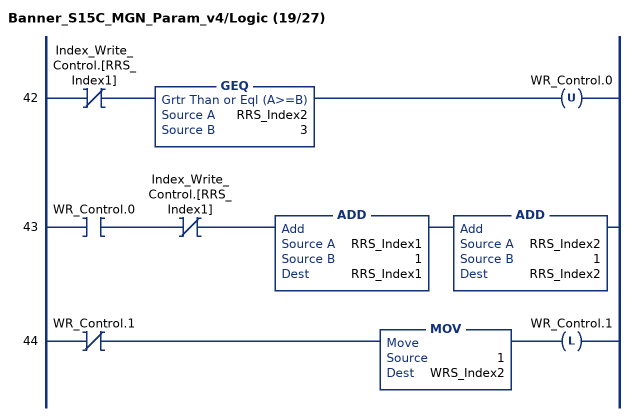
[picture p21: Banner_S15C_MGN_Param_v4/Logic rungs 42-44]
   42: XIO(Index_Write_Control.[RRS_Index1])GEQ(RRS_Index2,3)OTU(WR_Control.0);
   43: XIC(WR_Control.0)XIO(Index_Write_Control.[RRS_Index1])ADD(RRS_Index1,1,RRS_Index1)ADD(RRS_Index2,1,RRS_Index2);
   44: XIO(WR_Control.1)MOV(1,WRS_Index2)OTL(WR_Control.1);
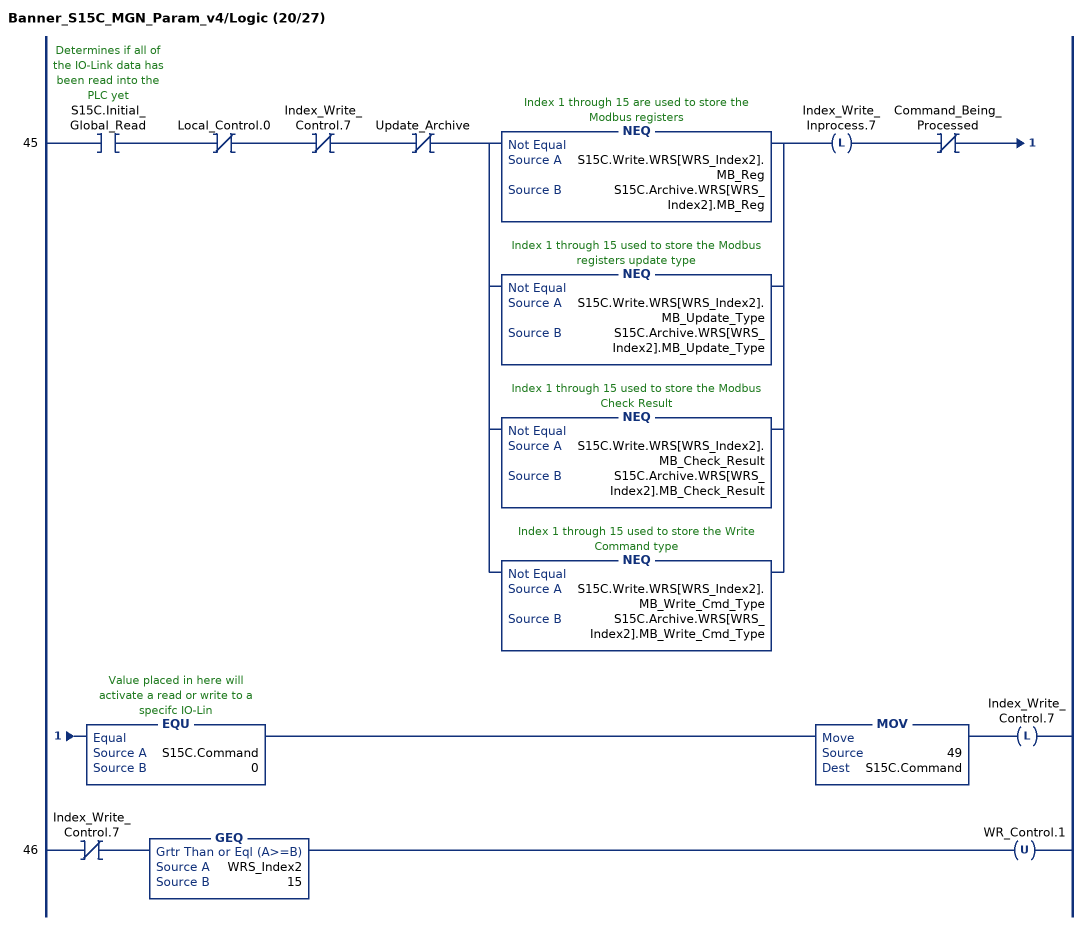
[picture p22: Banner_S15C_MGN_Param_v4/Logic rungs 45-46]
   45: XIC(S15C.Initial_Global_Read)XIO(Local_Control.0)XIO(Index_Write_Control.7)XIO(Update_Archive)[NEQ(S15C.Write.WRS[WRS_Index2].MB_Reg,S15C.Archive.WRS[WRS_Index2].MB_Reg) ,NEQ(S15C.Write.WRS[WRS_Index2].MB_Update_Type,S15C.Archive.WRS[WRS_Index2].MB_Update_Type) ,NEQ(S15C.Write.WRS[WRS_Index2].MB_Check_Result,S15C.Archive.WRS[WRS_Index2].MB_Check_Result) ,NEQ(S15C.Write.WRS[WRS_Index2].MB_Write_Cmd_Type,S15C.Archive.WRS[WRS_Index2].MB_Write_Cmd_Type) ]OTL(Index_Write_Inprocess.7)XIO(Command_Being_Processed)EQU(S15C.Command,0)MOV(49,S15C.Command)OTL(Index_Write_Control.7);
   46: XIO(Index_Write_Control.7)GEQ(WRS_Index2,15)OTU(WR_Control.1);
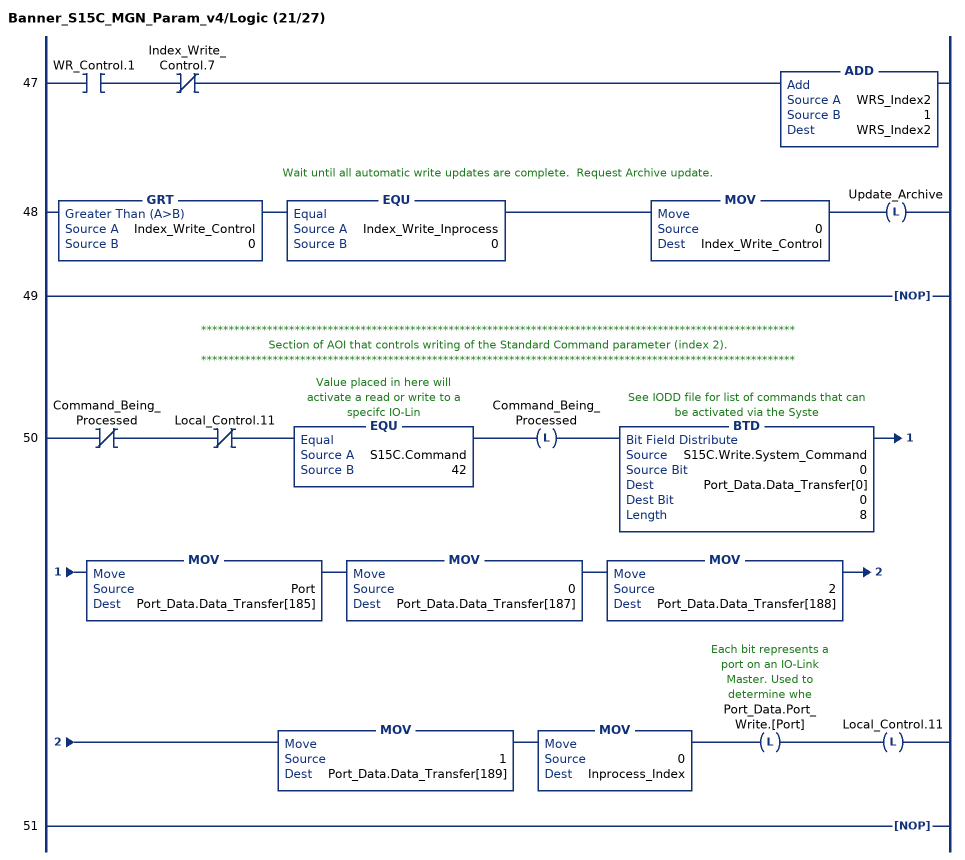
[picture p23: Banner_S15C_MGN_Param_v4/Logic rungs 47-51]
   47: XIC(WR_Control.1)XIO(Index_Write_Control.7)ADD(WRS_Index2,1,WRS_Index2);
   // Wait until all automatic write updates are complete.  Request Archive update.
   48: GRT(Index_Write_Control,0)EQU(Index_Write_Inprocess,0)MOV(0,Index_Write_Control)OTL(Update_Archive);
   49: NOP();
   // ************************************************************************************************************
   // Section of AOI that controls writing of the Standard Command parameter (index 2).
   // ************************************************************************************************************
   50: XIO(Command_Being_Processed)XIO(Local_Control.11)EQU(S15C.Command,42)OTL(Command_Being_Processed)BTD(S15C.Write.System_Command,0,Port_Data.Data_Transfer[0],0,8)MOV(Port,Port_Data.Data_Transfer[185])MOV(0,Port_Data.Data_Transfer[187])MOV(2,Port_Data.Data_Transfer[188])MOV(1,Port_Data.Data_Transfer[189])MOV(0,Inprocess_Index)OTL(Port_Data.Port_Write.[Port])OTL(Local_Control.11);
   51: NOP();
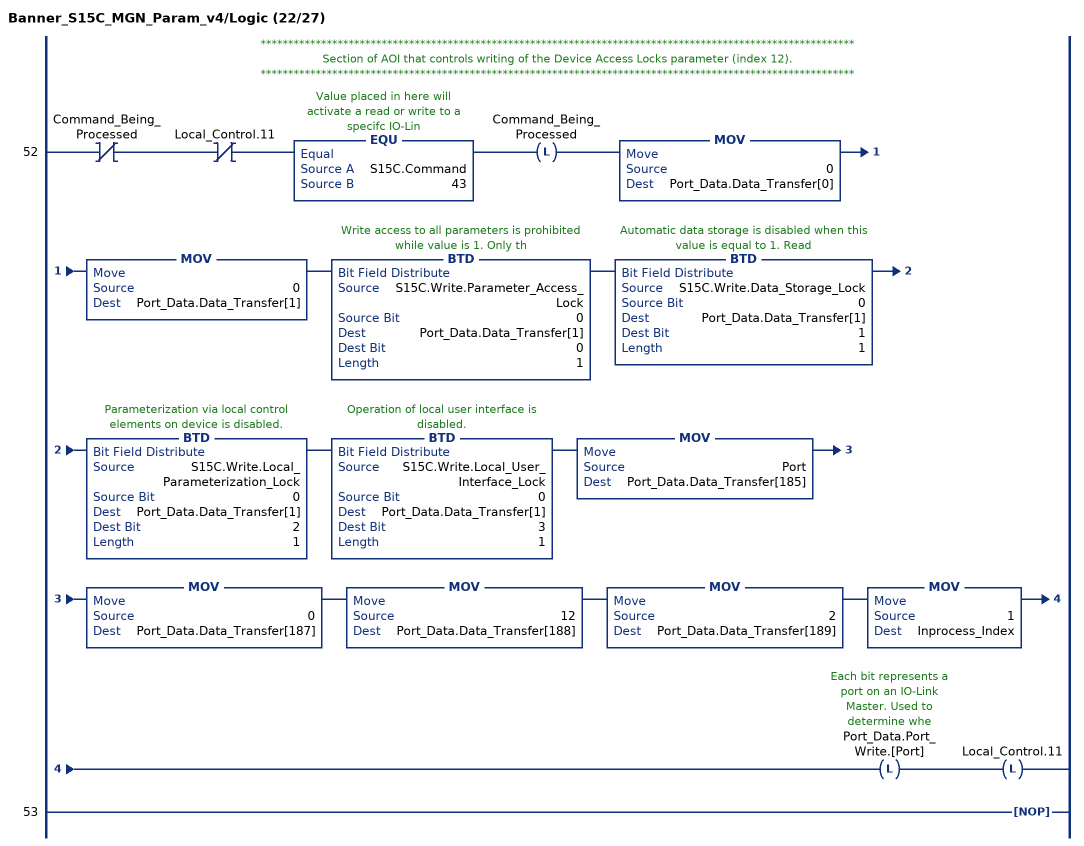
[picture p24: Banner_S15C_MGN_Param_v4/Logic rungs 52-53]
   // ************************************************************************************************************
   // Section of AOI that controls writing of the Device Access Locks parameter (index 12).
   // ************************************************************************************************************
   52: XIO(Command_Being_Processed)XIO(Local_Control.11)EQU(S15C.Command,43)OTL(Command_Being_Processed)MOV(0,Port_Data.Data_Transfer[0])MOV(0,Port_Data.Data_Transfer[1])BTD(S15C.Write.Parameter_Access_Lock,0,Port_Data.Data_Transfer[1],0,1)BTD(S15C.Write.Data_Storage_Lock,0,Port_Data.Data_Transfer[1],1,1)BTD(S15C.Write.Local_Parameterization_Lock,0,Port_Data.Data_Transfer[1],2,1)BTD(S15C.Write.Local_User_Interface_Lock,0,Port_Data.Data_Transfer[1],3,1)MOV(Port,Port_Data.Data_Transfer[185])MOV(0,Port_Data.Data_Transfer[187])MOV(12,Port_Data.Data_Transfer[188])MOV(2,Port_Data.Data_Transfer[189])MOV(1,Inprocess_Index)OTL(Port_Data.Port_Write.[Port])OTL(Local_Control.11);
   53: NOP();
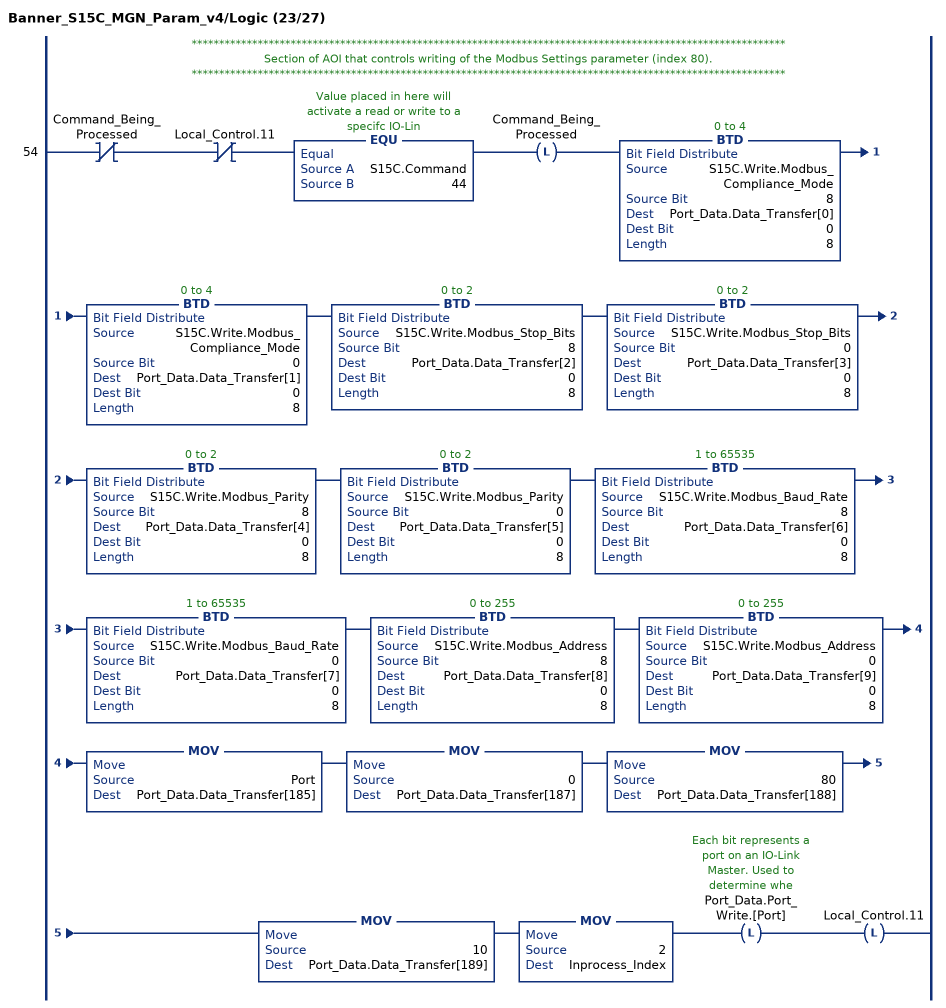
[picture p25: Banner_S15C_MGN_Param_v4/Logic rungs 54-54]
   // ************************************************************************************************************
   // Section of AOI that controls writing of the Modbus Settings parameter (index 80).
   // ************************************************************************************************************
   54: XIO(Command_Being_Processed)XIO(Local_Control.11)EQU(S15C.Command,44)OTL(Command_Being_Processed)BTD(S15C.Write.Modbus_Compliance_Mode,8,Port_Data.Data_Transfer[0],0,8)BTD(S15C.Write.Modbus_Compliance_Mode,0,Port_Data.Data_Transfer[1],0,8)BTD(S15C.Write.Modbus_Stop_Bits,8,Port_Data.Data_Transfer[2],0,8)BTD(S15C.Write.Modbus_Stop_Bits,0,Port_Data.Data_Transfer[3],0,8)BTD(S15C.Write.Modbus_Parity,8,Port_Data.Data_Transfer[4],0,8)BTD(S15C.Write.Modbus_Parity,0,Port_Data.Data_Transfer[5],0,8)BTD(S15C.Write.Modbus_Baud_Rate,8,Port_Data.Data_Transfer[6],0,8)BTD(S15C.Write.Modbus_Baud_Rate,0,Port_Data.Data_Transfer[7],0,8)BTD(S15C.Write.Modbus_Address,8,Port_Data.Data_Transfer[8],0,8)BTD(S15C.Write.Modbus_Address,0,Port_Data.Data_Transfer[9],0,8)MOV(Port,Port_Data.Data_Transfer[185])MOV(0,Port_Data.Data_Transfer[187])MOV(80,Port_Data.Data_Transfer[188])MOV(10,Port_Data.Data_Transfer[189])MOV(2,Inprocess_Index)OTL(Port_Data.Port_Write.[Port])OTL(Local_Control.11);
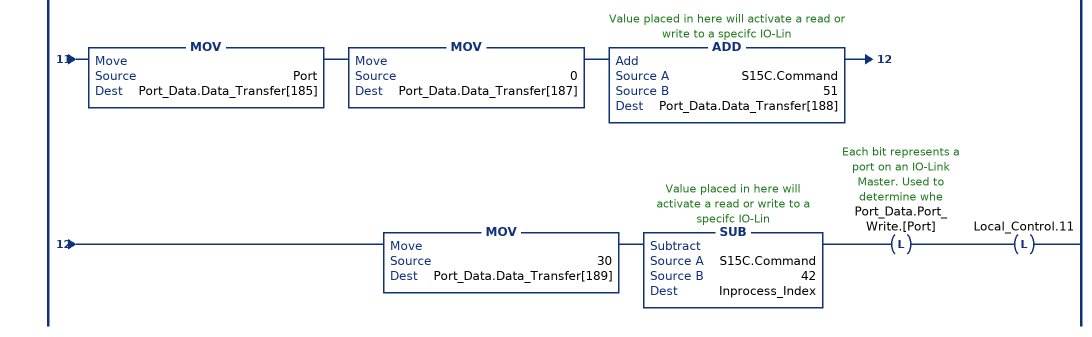
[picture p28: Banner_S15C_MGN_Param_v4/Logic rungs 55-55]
   // ************************************************************************************************************
   // Section of AOI that controls writing of the Read Registers Set 0 through 3 Settings parameter (index 96 to 99).
   // ************************************************************************************************************
   55: XIO(Command_Being_Processed)XIO(Local_Control.11)GEQ(S15C.Command,45)LEQ(S15C.Command,48)SUB(S15C.Command,45,RRS_Index3)OTL(Command_Being_Processed)BTD(S15C.Write.RRS[RRS_Index3].MB_Reg[15],8,Port_Data.Data_Transfer[0],0,8)BTD(S15C.Write.RRS[RRS_Index3].MB_Reg[15],0,Port_Data.Data_Transfer[1],0,8)BTD(S15C.Write.RRS[RRS_Index3].MB_Reg[14],8,Port_Data.Data_Transfer[2],0,8)BTD(S15C.Write.RRS[RRS_Index3].MB_Reg[14],0,Port_Data.Data_Transfer[3],0,8)BTD(S15C.Write.RRS[RRS_Index3].MB_Reg[13],8,Port_Data.Data_Transfer[4],0,8)BTD(S15C.Write.RRS[RRS_Index3].MB_Reg[13],0,Port_Data.Data_Transfer[5],0,8)BTD(S15C.Write.RRS[RRS_Index3].MB_Reg[12],8,Port_Data.Data_Transfer[6],0,8)BTD(S15C.Write.RRS[RRS_Index3].MB_Reg[12],0,Port_Data.Data_Transfer[7],0,8)BTD(S15C.Write.RRS[RRS_Index3].MB_Reg[11],8,Port_Data.Data_Transfer[8],0,8)BTD(S15C.Write.RRS[RRS_Index3].MB_Reg[11],0,Port_Data.Data_Transfer[9],0,8)BTD(S15C.Write.RRS[RRS_Index3].MB_Reg[10],8,Port_Data.Data_Transfer[10],0,8)BTD(S15C.Write.RRS[RRS_Index3].MB_Reg[10],0,Port_Data.Data_Transfer[11],0,8)BTD(S15C.Write.RRS[RRS_Index3].MB_Reg[9],8,Port_Data.Data_Transfer[12],0,8)BTD(S15C.Write.RRS[RRS_Index3].MB_Reg[9],0,Port_Data.Data_Transfer[13],0,8)BTD(S15C.Write.RRS[RRS_Index3].MB_Reg[8],8,Port_Data.Data_Transfer[14],0,8)BTD(S15C.Write.RRS[RRS_Index3].MB_Reg[8],0,Port_Data.Data_Transfer[15],0,8)BTD(S15C.Write.RRS[RRS_Index3].MB_Reg[7],8,Port_Data.Data_Transfer[16],0,8)BTD(S15C.Write.RRS[RRS_Index3].MB_Reg[7],0,Port_Data.Data_Transfer[17],0,8)BTD(S15C.Write.RRS[RRS_Index3].MB_Reg[6],8,Port_Data.Data_Transfer[18],0,8)BTD(S15C.Write.RRS[RRS_Index3].MB_Reg[6],0,Port_Data.Data_Transfer[19],0,8)BTD(S15C.Write.RRS[RRS_Index3].MB_Reg[5],8,Port_Data.Data_Transfer[20],0,8)BTD(S15C.Write.RRS[RRS_Index3].MB_Reg[5],0,Port_Data.Data_Transfer[21],0,8)BTD(S15C.Write.RRS[RRS_Index3].MB_Reg[4],8,Port_Data.Data_Transfer[22],0,8)BTD(S15C.Write.RRS[RRS_Index3].MB_Reg[4],0,Port_Data.Data_Transfer[23],0,8)BTD(S15C.Write.RRS[RRS_Index3].MB_Reg[3],8,Port_Data.Data_Transfer[24],0,8)BTD(S15C.Write.RRS[RRS_Index3].MB_Reg[3],0,Port_Data.Data_Transfer[25],0,8)BTD(S15C.Write.RRS[RRS_Index3].MB_Reg[2],8,Port_Data.Data_Transfer[26],0,8)BTD(S15C.Write.RRS[RRS_Index3].MB_Reg[2],0,Port_Data.Data_Transfer[27],0,8)BTD(S15C.Write.RRS[RRS_Index3].MB_Reg[1],8,Port_Data.Data_Transfer[28],0,8)BTD(S15C.Write.RRS[RRS_Index3].MB_Reg[1],0,Port_Data.Data_Transfer[29],0,8)MOV(Port,Port_Data.Data_Transfer[185])MOV(0,Port_Data.Data_Transfer[187])ADD(S15C.Command,51,Port_Data.Data_Transfer[188])MOV(30,Port_Data.Data_Transfer[189])SUB(S15C.Command,42,Inprocess_Index)OTL(Port_Data.Port_Write.[Port])OTL(Local_Control.11);
